{attribute 'no_assign'}
FUNCTION_BLOCK FB_DO_IED_MUnn_LPHD1_Proxy EXTENDS FB_AcsiCommonDataClass
VAR_INPUT
	stVal: FB_AcsiBATypeBOOLEAN := (Fc:=ACSI_FC_ST, TrgOp:=ACSI_TrgOp_dchg, bLinkResult:=THIS^.AddDataToContainer(ipData:=stVal));
	q: FB_AcsiDATypeQuality := (Fc:=ACSI_FC_ST, TrgOp:=ACSI_TrgOp_qchg, bLinkResult:=THIS^.AddDataToContainer(ipData:=q));
	t: FB_AcsiDATypeTimeStamp := (Fc:=ACSI_FC_ST, bLinkResult:=THIS^.AddDataToContainer(ipData:=t));
END_VAR
VAR
END_VAR

END_FUNCTION_BLOCK
